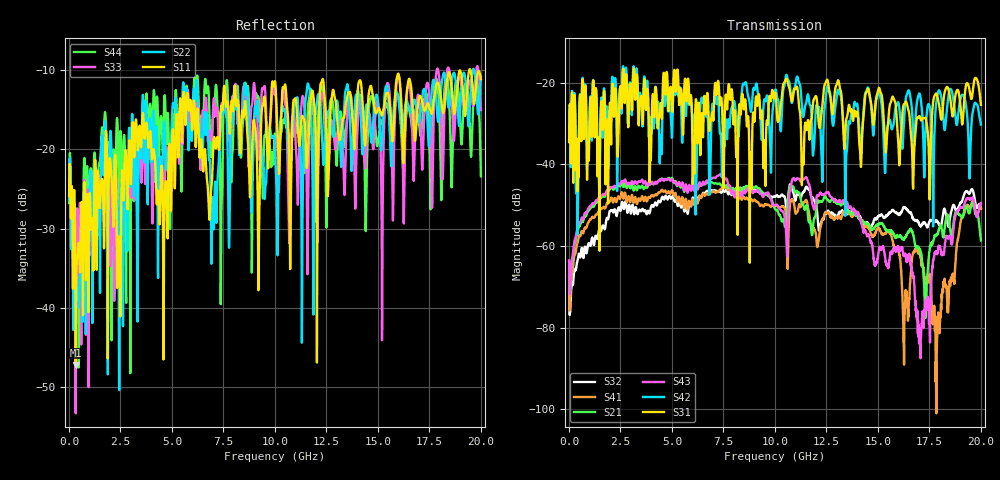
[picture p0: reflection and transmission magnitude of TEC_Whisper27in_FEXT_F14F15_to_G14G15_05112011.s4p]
! Tyco Electronics
! F14F15-G14G15_FEXT
!! PART DESCRIPTION: Whisper 27in Megtron 6 VLP-HVLP-VLP Channel Model, bulkhead 2.4mm test pts
!! MODEL DESCRIPTION: System 4-port S-parameter
!! MODEL STATUS: Measured
!! MODEL GEOMETRY: Channel Model
!! MODEL FREQUENCY RANGE: DC to 20.000 GHz in 10.000 MHz frequency steps
!! MODEL EDGE RATE LIMITATION: 25.50 ps (Using conservative 0.5/Fmax rule of thumb)
!! TIME-DOMAIN TRANSFORM CAUTIONS:
!! 1.) Do not simulate transient edge rates faster than the number listed above.  Edge rates faster than this number
!!  contain significant spectral content at frequencies above the model's highest frequency.
!! 2.) Even when simulating edge rates that are slower than the number listed above, be aware that the best time
!!  resolution possible with a direct iFFT is (1 / 2Fmax).  As a result, time resolution is typically not adequate
!!  for most time-domain simulations unless tricks such as windowing are used to minimize leakage and aliasing.
!! 3.) Because the model has a uniform frequency step, a direct iFFT will result in an impulse that that has a time
!!  length given by either (1 / Fstep) or (1 / 2Fstep), depending on the transform being used.  Care has been taken
!!  in selecting the frequency step to ensure a settled impulse response for the model.  Therefore, convolution with
!!  the model's impulse response should present no issues.  However, if directly concatenating s-parameter models
!!  in the frequency domain a user must either interpolate necessary interim frequencies or complete impulse response
!!  zero-padding.  Impulse response zero-padding is more difficult, but more accurate.
!! PORT DEFINITIONS:
!! Port  1  ----->  Side A  F14  G14  Side B  <-----  Port  2
!! Port  3  ----->  Side A  F15  G15  Side B  <-----  Port  4
! Point-to-Point link (differential)  !
! Connectors:  !
!  1: STRADA Whisper  !
! Materials:  !
!  Backplane: Megtron-6 HVLP  !
!  Daughtercard: Megtron-6 VLP  !
! Stack-up:  !
!  Backplane: 20 layers, 200mil thick  !
!  Daughtercard: 14 layers, 110mil thick  !
! Trace Length:  !
!  Backplane: 17in  !
!  Daightercards: 5in  !
! Trace Width:  !
!  Backplane: 8-13-8 mils  !
!  Daughtercards: 6-9-6 mils  !
! Geometry:  !
!  Backplane: Stripline  !
!  Daughtercards: Stripline  !
! Freq. Range: 0 GHz - 20 GHz  !
! Note1: non-mixed-mode s-parameters  !
! Note2: channel includes 2.4mm test points  !
! Created Wed May 11 14:42:47 2011
! 4 Port Network Data from SP1.SP block
! freq  magS11  angS11  magS12  angS12  magS13  angS13  magS14  angS14
!  magS21  angS21  magS22  angS22  magS23  angS23  magS24  angS24
!  magS31  angS31  magS32  angS32  magS33  angS33  magS34  angS34
!  magS41  angS41  magS42  angS42  magS43  angS43  magS44  angS44
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# hz S ma R 50
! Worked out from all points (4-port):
!   2000 points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, 10 MHz to 20 GHz, reference 50 ohm
!   strongest paths, dB at 10 MHz, 5.01 GHz, 10.01 GHz, 15.01 GHz, 20 GHz:
!     S31: -34.6, -25.9, -22.5, -21.9, -25.5
!     S42: -34.6, -33.2, -21.9, -22.4, -30.3
!     S43: -63.5, -43.6, -50.0, -62.5, -49.6
!     S21: -63.8, -43.3, -51.0, -54.9, -58.7
!     S41: -67.6, -46.4, -50.2, -55.7, -50.8
!     S32: -67.1, -47.9, -47.9, -52.8, -50.9
!   lowest |S11| = -47.1 dB at 330 MHz (marker M1), VSWR 1.01, Z = 49.6 - j0.02 ohm
!   |S11| at or under -10 dB: start of sweep to 19.44 GHz; 19.49 GHz to end of sweep
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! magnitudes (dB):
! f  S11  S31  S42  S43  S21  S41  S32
! 10 MHz  -25.9  -34.6  -34.6  -63.5  -63.8  -67.6  -67.1
! 330 MHz  -47.1  -38.3  -35.6  -57.8  -58.6  -61.5  -65.6
! 11.48 GHz  -18.1  -29.8  -25.5  -43.4  -50.8  -49.0  -45.8
! 16.28 GHz  -20.0  -25.2  -28.6  -62.3  -58.3  -79.7  -50.5
! 17.03 GHz  -13.3  -28.3  -22.8  -81.2  -61.1  -61.8  -54.9
! 17.89 GHz  -11.6  -23.4  -23.1  -61.7  -57.1  -77.3  -54.1
! 20 GHz  -11.1  -25.5  -30.3  -49.6  -58.7  -50.8  -50.9
